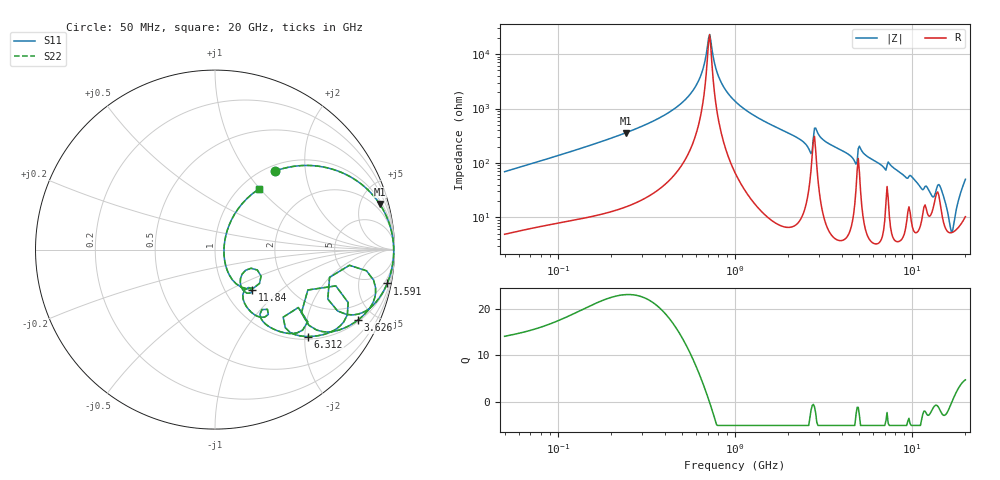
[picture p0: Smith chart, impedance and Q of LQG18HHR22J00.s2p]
!Murata Part Number: LQG18HHR22J00
!These Parameters are Measured in Series Mode Connection
!  o--[Z]--o
!Port1  Port2
!  o-------o
!Freq. Start=50[MHz] Stop=20[GHz], 401[Steps]
# Hz S RI R 50
!Freq.(Hz) S11(Real) S11(Imag) S21(Real) S21(Imag) S12(Real) S12(Imag) S22(Real) S22(Imag)
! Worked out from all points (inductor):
!   401 points, 50 MHz to 20 GHz, reference 50 ohm
!   read as one part in series: L = 216 nH near 51.52 MHz
!   highest Q = 23 at 241 MHz (marker M1), where L = 235 nH
!   self-resonance near 708.6 MHz
!   S11 on the Smith chart (normalised r, x): 50 MHz: 1.10, +1.38; 1.591 GHz: 1, -10; 3.626 GHz: 1.08, -4.01; 6.312 GHz: 1.07, -2.08; 11.84 GHz: 1.34, -0.66; 20 GHz: 1.21, +0.98
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5e7  0.3343 0.4375  0.6657 -0.4375  0.6657 -0.4375  0.3343 0.4375
1.364002e8  0.7679 0.3976  0.2321 -0.3976  0.2321 -0.3976  0.7679 0.3976
2.409965e8  0.9177 0.2539  0.0823 -0.2539  0.0823 -0.2539  0.9177 0.2539
3.721004e8  0.9711 0.1447  0.0289 -0.1447  0.0289 -0.1447  0.9711 0.1447
5.831961e8  0.993 0.0442  0.00698 -0.0442  0.00698 -0.0442  0.993 0.0442
6.476653e8  0.9949 0.0218  0.00512 -0.0218  0.00512 -0.0218  0.9949 0.0218
7.192613e8  0.9957 -0.000471  0.00432 0.000471  0.00432 0.000471  0.9957 -0.000471
8.230629e8  0.9952 -0.0294  0.00483 0.0294  0.00483 0.0294  0.9952 -0.0294
1e9  0.9912 -0.0724  0.00885 0.0724  0.00885 0.0724  0.9912 -0.0724
1.590961e9  0.9595 -0.1884  0.0405 0.1884  0.0405 0.1884  0.9595 -0.1884
2.531158e9  0.8 -0.3587  0.2 0.3587  0.2 0.3587  0.8 -0.3587
2.728004e9  0.6382 -0.1546  0.3618 0.1546  0.3618 0.1546  0.6382 -0.1546
2.853386e9  0.8834 -0.1698  0.1166 0.1698  0.1166 0.1698  0.8834 -0.1698
3.626126e9  0.7962 -0.3925  0.2038 0.3925  0.2038 0.3925  0.7962 -0.3925
4.539627e9  0.6237 -0.4589  0.3763 0.4589  0.3763 0.4589  0.6237 -0.4589
4.966507e9  0.6733 -0.2022  0.3267 0.2022  0.3267 0.2022  0.6733 -0.2022
6.311513e9  0.5186 -0.4842  0.4814 0.4842  0.4814 0.4842  0.5186 -0.4842
7.442007e9  0.4882 -0.4487  0.5118 0.4487  0.5118 0.4487  0.4882 -0.4487
1.183995e10  0.2084 -0.2236  0.7916 0.2236  0.7916 0.2236  0.2084 -0.2236
1.460232e10  0.1773 -0.2183  0.8227 0.2183  0.8227 0.2183  0.1773 -0.2183
1.670968e10  0.0499 -0.00687  0.9501 0.00687  0.9501 0.00687  0.0499 -0.00687
2e10  0.2431 0.3364  0.7569 -0.3364  0.7569 -0.3364  0.2431 0.3364
